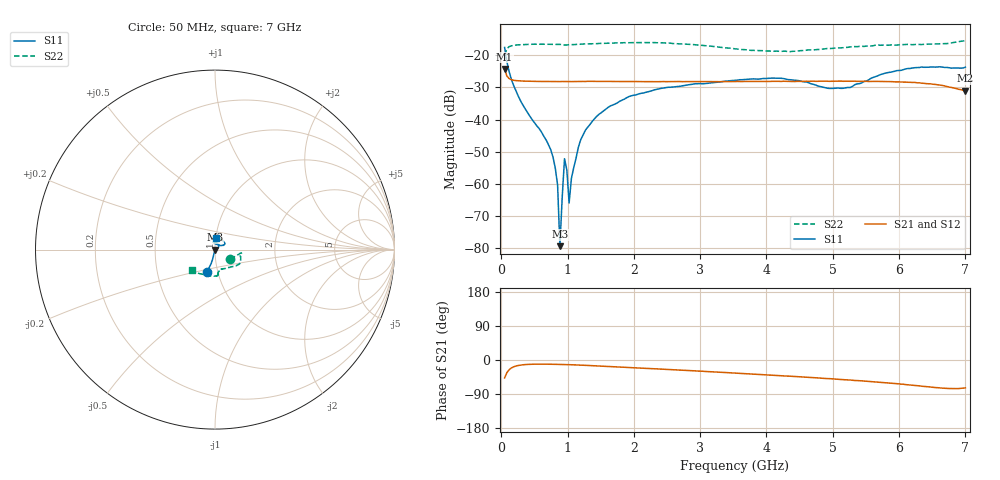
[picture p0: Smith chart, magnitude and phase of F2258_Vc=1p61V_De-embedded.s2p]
! Integrated Device Technology
! Corporate Headquarters
! 6024 Silver Creek Valley Road
! San Jose, CA 95138  USA
! Phone:  1-408-284-8200
! Toll Free:  1-800-223-1366
! Webpage:  http://www.idt.com/
! Timing and RF Division
! 515 Groton Road, Suite 102
! Westford, MA 01886-6024
! Device:  F2258
! Description: Voltage Variable RF Attenuator
! Frequency:  50.0 -  6000.00 MHz
! Package:  3x3 mm Thin QFN Plastic Package: 16 pin
! Ports:  2 RF, 2 DC
!  Pin  1  = NC
!  Pin  2  = NC
!  Pin  3  = RF2  = Port 2
!  Pin  4  = GND
!  Pin  5  = Vdd
!  Pin  6  = NC
!  Pin  7  = VCTRL
!  Pin  8  = NC
!  Pin  9  = GND
!  Pin 10  = RF1  = Port 1
!  Pin 11  = NC
!  Pin 12  = NC
!  Pin 13  = NC
!  Pin 14  = NC
!  Pin 15  = NC
!  Pin 16  = NC
! Vcntrl:  1.610 Volts
! Vdd:  +3.300 Volts
! Current:  1.161 mA
! Data:  The device was measured on a the F2258 evaluation board which has
!  individual transmission lines to the RF pins.  Data was collected
!  using a calibrated network analyzer.  The evaluation board was
!  de-embedded using a TRL calibration technique.
!  The reference plane is the edge of the package pin.
! Misc:  SN 10
!  Action Tracker AT0285
! Date Measured:  2014-12-10
! Date:  2016-01-13  MJV
! Note:
!  Integrated Device Technology supplies this data as a sample of measured
!  data at the package pin for this product.  Your particular data for this
!  product may vary.
!  Data was taken at 25 degrees C.
!  Integrated Device Technology reserves the right to change this data at anytime.
!Freq_(GHz)  S11M_(dB)  S11P_(deg)  S21M_(dB)  S21P_(deg)  S12M_(dB)  S12P_(deg)  S22M_(dB)  S22P_(deg)
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# GHz S dB R 50
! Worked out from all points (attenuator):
!   201 points, 50 MHz to 7 GHz, reference 50 ohm
!   highest |S21| = -24.27 dB at 50 MHz (marker M1); lowest = -31.0 dB at 7 GHz (marker M2)
!   lowest |S11| = -79.5 dB at 884 MHz (marker M3), VSWR 1.00, Z = 50 - j0.00851 ohm
!   |S11| at or under -10 dB: start of sweep to end of sweep
!   |S22| runs from -20.0 to -15.3 dB; largest |S21 - S12| = 0.00032
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0.05  -17.54 -109.5  -24.27 -47.1  -24.26 -47.1  -20.01 -32.3
0.1195  -25.15 -104.0  -27.24 -25.5  -27.23 -25.5  -17.26 -10.0
0.22375  -31.18 -105.3  -27.86 -15.8  -27.87 -15.8  -16.77 -6.8
0.6755  -46.34 -104.2  -28.12 -11.0  -28.19 -11.0  -16.51 -10.1
0.77975  -51.66 -107.8  -28.15 -11.3  -28.16 -11.3  -16.54 -11.6
0.84925  -60.42 -102.5  -28.16 -11.5  -28.16 -11.5  -16.57 -12.6
0.884  -79.46 -53.1  -28.16 -11.7  -28.15 -11.7  -16.58 -13.4
0.91875  -64.25 60.6  -28.14 -11.9  -28.17 -11.9  -16.60 -13.9
0.9535  -52.20 -128.8  -28.15 -12.0  -28.17 -12.0  -16.78 -13.6
0.98825  -55.65 -138.0  -28.16 -12.2  -28.17 -12.2  -16.76 -14.4
1.023  -66.00 -84.5  -28.18 -12.4  -28.18 -12.4  -16.69 -14.9
1.05775  -58.29 -8.3  -28.17 -12.6  -28.17 -12.5  -16.65 -15.2
1.162  -48.67 26.7  -28.13 -13.2  -28.16 -13.2  -16.53 -16.7
1.2315  -44.86 22.1  -28.12 -13.7  -28.15 -13.7  -16.46 -17.6
1.6485  -35.72 25.1  -28.11 -17.5  -28.16 -17.4  -16.18 -22.7
2.37825  -30.41 43.5  -28.20 -23.7  -28.21 -23.7  -16.06 -31.2
3.525  -27.80 89.4  -28.15 -34.5  -28.14 -34.5  -17.95 -51.6
4.1505  -27.06 104.0  -28.09 -40.8  -28.10 -40.8  -18.66 -69.3
4.7065  -29.02 94.4  -28.04 -46.5  -28.02 -46.6  -18.29 -79.5
5.2625  -30.02 51.1  -28.06 -52.8  -28.07 -52.8  -17.35 -82.9
5.85325  -25.30 27.7  -28.18 -61.0  -28.20 -61.0  -16.82 -83.8
7  -23.67 83.7  -30.97 -73.6  -30.98 -73.6  -15.35 -137.4
